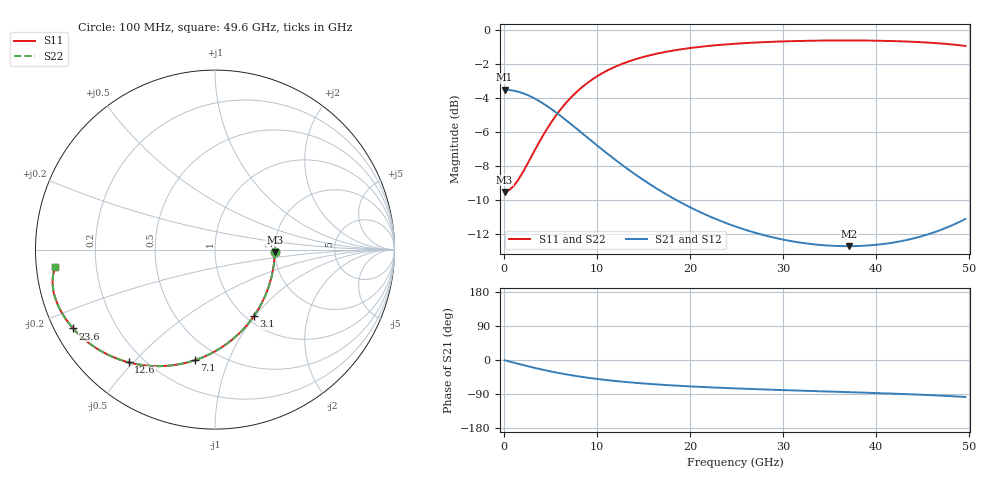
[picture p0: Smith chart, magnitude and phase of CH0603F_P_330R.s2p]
# GHz S RI R 330
! S-Parameters data
! Freq  reS11  imS11  reS21  imS21  reS12  imS12  reS22  imS22
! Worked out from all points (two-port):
!   100 points, 100 MHz to 49.6 GHz, reference 330 ohm
!   highest |S21| = -3.52 dB at 100 MHz (marker M1); lowest = -12.7 dB at 37.1 GHz (marker M2)
!   |S21| within 3 dB of the highest: start of sweep to 9.41 GHz
!   lowest |S11| = -9.5 dB at 100 MHz (marker M3), VSWR 2.00, Z = 659 - j19.6 ohm
!   |S11| at or under -10 dB: nowhere
!   |S22| runs from -9.5 to -0.6 dB; largest |S21 - S12| = 0
!   S11 on the Smith chart (normalised r, x): 100 MHz: 2.00, -0.06; 3.1 GHz: 1.08, -0.99; 7.1 GHz: 0.37, -0.76; 12.6 GHz: 0.14, -0.49; 23.6 GHz: 0.05, -0.26; 49.6 GHz: 0.06, -0.06
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0.1  0.3332 -0.0132  0.6666 -0.00755  0.6666 -0.00755  0.3332 -0.0132
0.6  0.3285 -0.0788  0.6638 -0.0451  0.6638 -0.0451  0.3285 -0.0788
1.6  0.2999 -0.2055  0.6465 -0.1174  0.6465 -0.1174  0.2999 -0.2055
3.1  0.2162 -0.3719  0.5966 -0.2106  0.5966 -0.2106  0.2162 -0.3719
4.1  0.1412 -0.461  0.5527 -0.2591  0.5527 -0.2591  0.1412 -0.461
5.1  0.058 -0.5307  0.505 -0.2958  0.505 -0.2958  0.058 -0.5307
6.1  -0.028 -0.5819  0.4566 -0.3216  0.4566 -0.3216  -0.028 -0.5819
7.1  -0.1128 -0.6167  0.41 -0.3381  0.41 -0.3381  -0.1128 -0.6167
8.6  -0.2321 -0.6439  0.3463 -0.3495  0.3463 -0.3495  -0.2321 -0.6439
10.6  -0.3697 -0.6472  0.2756 -0.3483  0.2756 -0.3483  -0.3697 -0.6472
12.6  -0.4814 -0.628  0.2204 -0.3373  0.2204 -0.3373  -0.4814 -0.628
14.6  -0.5702 -0.5974  0.1779 -0.3224  0.1779 -0.3224  -0.5702 -0.5974
16.6  -0.6403 -0.5621  0.1451 -0.3067  0.1451 -0.3067  -0.6403 -0.5621
19.6  -0.7191 -0.5076  0.1091 -0.2848  0.1091 -0.2848  -0.7191 -0.5076
23.6  -0.7903 -0.4392  0.0766 -0.2612  0.0766 -0.2612  -0.7903 -0.4392
25.1  -0.8101 -0.4155  0.0675 -0.2542  0.0675 -0.2542  -0.8101 -0.4155
28.6  -0.846 -0.3642  0.0502 -0.2414  0.0502 -0.2414  -0.846 -0.3642
33.1  -0.8767 -0.3051  0.0333 -0.2321  0.0333 -0.2321  -0.8767 -0.3051
37.1  -0.8939 -0.2568  0.0205 -0.2303  0.0205 -0.2303  -0.8939 -0.2568
41.6  -0.9037 -0.2038  0.00576 -0.2363  0.00576 -0.2363  -0.9037 -0.2038
45.6  -0.9035 -0.1546  -0.0108 -0.2503  -0.0108 -0.2503  -0.9035 -0.1546
49.6  -0.8905 -0.0991  -0.0366 -0.2756  -0.0366 -0.2756  -0.8905 -0.0991
